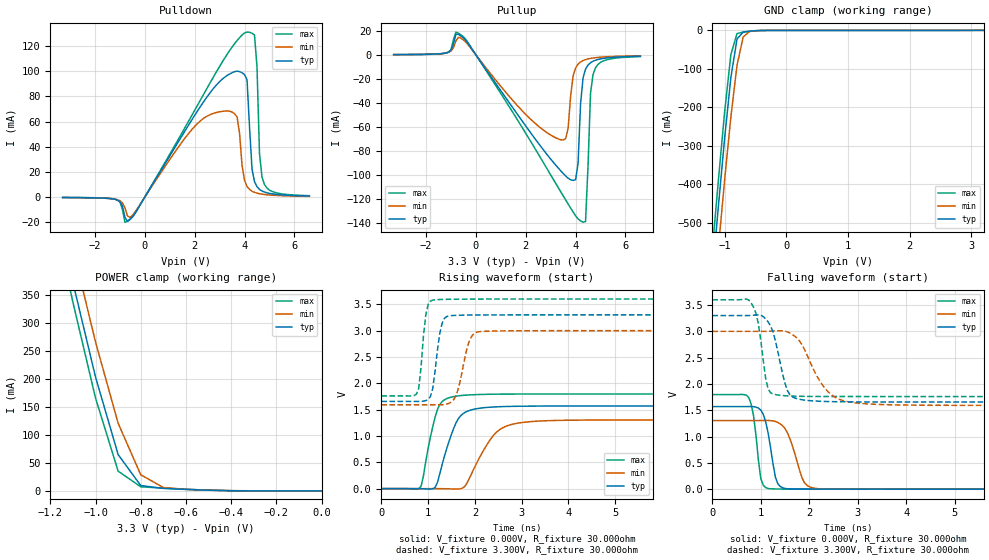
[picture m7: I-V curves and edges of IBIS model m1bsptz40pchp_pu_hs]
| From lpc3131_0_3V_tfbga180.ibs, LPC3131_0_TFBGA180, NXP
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| |   Rev 0.20 IBIS Model Design Automation Generation   |
| |   N O N - S I L I C O N   C O R R E L A T E D   |
| |   This IBIS [Model] is pre-Beta tactical support   |
| |  Note: this IBIS [Model] contains clamp curves generated   |
| |   through simulation which should not be relied upon   |
| Date/Time   : 2010 Jan 25 (Mon) 11:58:19
| Pccmos090 jliolib_p50 2.0
|   0.9 um 3.3V pad library
|   seven level metal
|   dual oxide
|   dual threshold voltage
|   nominal line mixed supply
|   parasitic extracted netlists
| Process block a10
| mem1bsptz40pchp
|   Bidirectional Pad 3.3
|   3state Output
|   Plain Input
|   CMOS
|   Programmable between
|   - (p1=0, p2=1) plain input
|   - (p1=0, p2=0) with Pull Up
|   - (p1=1, p2=1) with Pull Down
|   - (p1=1, p2=0) with Repeater
| Pull Up Mode high speed (esh=0, p1=0, p2=0)
[Model]   m1bsptz40pchp_pu_hs | of mem1bsptz40pchp
Model_type   I/O
Polarity   Non-Inverting
Enable   Active-Low
|  Reciever Thresholds
Vinl   = 0.99V
Vinh   = 2.31V
| AC Test Load Conditions
Vref   = 0
Cref   = 0
Rref   = 1000000000
Vmeas   = 1.65
| [Process Range]   typical   min   max
| C_comp edge width   400.000ps   400.000ps   400.000ps
| C_comp Tstrobe   40.000fs   40.000fs   40.000fs
C_comp   200.000pF   200.000pF   200.000pF
[Temperature Range]   25   125   -40
[Voltage Range]   3.30V   3.00V   3.60V
[GND Clamp Reference]   0.00V   0.00V   0.00V
[Pulldown Reference]   0.00V   0.00V   0.00V
[POWER Clamp Reference]   3.30V   3.00V   3.60V
[Pullup Reference]   3.30V   3.00V   3.60V
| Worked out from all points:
|   slope of the pulldown table from 0 to 0.495 V, typ, clamps not added: 30.7 ohm
|   slope of the pullup table from 0 to 0.495 V, typ, clamps not added: 33.4 ohm
|   GND clamp passes 1 mA (typ) near -0.51 V on its own axis
|   POWER clamp passes 1 mA (typ) near -0.47 V on its own axis
|   rising waveform, V_fixture 0.000V, R_fixture 30.000ohm: 20-80 % time 341ps typ, 514ps min, 255ps max; typ from 0.001 V to 1.57 V
|   falling waveform, V_fixture 0.000V, R_fixture 30.000ohm: 20-80 % time 178ps typ, 272ps min, 137ps max; typ from 1.57 V to 0.001 V
|   rising waveform, V_fixture 3.300V, R_fixture 30.000ohm: 20-80 % time 144ps typ, 213ps min, 115ps max; typ from 1.66 V to 3.3 V
|   falling waveform, V_fixture 3.300V, R_fixture 30.000ohm: 20-80 % time 251ps typ, 501ps min, 169ps max; typ from 3.3 V to 1.66 V
[GND Clamp]
| ref voltage   0.00V   0.00V   0.00V
|   Voltage   I(typ)   I(min)   I(max)
-3.3V     -4.732A    -4.814A    -4.684A
-1.2V     -636mA     -742.5mA   -569.7mA
-1.1V     -453.5mA   -561.8mA   -385.7mA
-1V       -279mA     -387.5mA   -210.8mA
-900mV    -122.8mA   -225.5mA   -63.15mA
-800mV    -22.47mA   -90.5mA    -8.27mA
-700mV    -4.437mA   -17.32mA   -4.624mA
-600mV    -2.227mA   -3.085mA   -2.65mA
-300mV    -253.1uA   -168.6uA   -385.4uA
3.2V      -17.82uA   34.39uA    -87.56uA
[Power Clamp]   | Vtable = Vcc - Vpad
| ref voltage   3.30V   3.00V   3.60V
|   Voltage   I(typ)   I(min)   I(max)
-3.3V     4.647A     4.675A     4.636A
-1.2V     553.3mA    610.4mA    520.8mA
-1.1V     373.2mA    433.6mA    337.9mA
-1V       204mA      266.6mA    166.4mA
-900mV    65.07mA    121.2mA    35.4mA
-800mV    9.632mA    28.93mA    7.456mA
-700mV    4.576mA    6.079mA    4.901mA
-600mV    2.711mA    2.826mA    2.897mA
-400mV    366.5uA    549.1uA    304.5uA
0V        388.1pA    9.875nA    264.4pA
[Pulldown]
| ref voltage   0.00V   0.00V   0.00V
|   Voltage   I(typ)   I(min)   I(max)
-3.3V     -237uA     -253uA     -192.2uA
-1.2V     -1.654mA   -1.559mA   -1.497mA
-600mV    -17.52mA   -16.02mA   -17.7mA
2.8V      87.36mA    66.79mA    96.99mA
3.7V      99.96mA    63.73mA    124.2mA
4.1V      93mA       8.514mA    130.9mA
4.3V      22.4mA     4.741mA    130.1mA
4.4V      12.38mA    3.859mA    128.6mA
4.5V      8.362mA    3.243mA    103.4mA
4.6V      6.217mA    2.791mA    34.69mA
4.8V      4.107mA    2.175mA    10.04mA
6.6V      975.1uA    710.1uA    1.215mA
[Pullup]   | Vtable = Vcc - Vpad
| ref voltage   3.30V   3.00V   3.60V
|   Voltage   I(typ)   I(min)   I(max)
-3.3V     206.8uA    209.1uA    174.1uA
-500mV    14.05mA    12.42mA    15mA
3.4V      -96.4mA    -70.68mA   -113.8mA
3.7V      -102.7mA   -61.31mA   -124.1mA
3.9V      -104.5mA   -17.66mA   -130.8mA
4.1V      -90.31mA   -7.691mA   -136.5mA
4.2V      -40.65mA   -5.885mA   -138.2mA
4.3V      -19.22mA   -4.74mA    -139.3mA
4.4V      -11.93mA   -3.955mA   -138.7mA
4.6V      -6.527mA   -2.958mA   -31.83mA
4.7V      -5.3mA     -2.623mA   -16.4mA
6.6V      -1.122mA   -812.7uA   -1.418mA
[Ramp]
R_load   = 30.000ohm
|   dV/dt(typ)   dV/dt(min)   dV/dt(max)
dV/dt_r   941.416mV/350.000ps   782.862mV/500.000ps   1.078V/250.000ps
dV/dt_f   985.623mV/250.000ps   844.107mV/500.000ps   1.103V/150.000ps
[Rising Waveform]  | cubic spline decimation from 501 points
V_fixture   = 0.000V
R_fixture   = 30.000ohm
|   Time   V(typ)   V(min)   V(max)
0s        906.1uV    713.4uV    1.177mV
850ps     -657.1uV   736.3uV    46.19mV
1.15ns    25.24mV    854.7uV    1.359V
1.3ns     457.5mV    -208.2uV   1.654V
1.55ns    1.154V     -5.889mV   1.749V
1.8ns     1.454V     61.17mV    1.776V
2.2ns     1.538V     751mV      1.79V
2.45ns    1.553V     1.063V     1.794V
3.3ns     1.568V     1.28V      1.797V
25ns      1.57V      1.305V     1.798V
[Falling Waveform]  | cubic spline decimation from 501 points
V_fixture   = 0.000V
R_fixture   = 30.000ohm
|   Time   V(typ)   V(min)   V(max)
0s        1.57V      1.305V     1.798V
750ps     1.571V     1.305V     1.742V
850ps     1.569V     1.305V     1.395V
1ns       1.504V     1.306V     198.2mV
1.2ns     794.7mV    1.304V     7.889mV
1.3ns     230.7mV    1.287V     5.057mV
1.4ns     53.05mV    1.243V     3.511mV
1.9ns     2.346mV    124.6mV    1.427mV
2.2ns     1.395mV    8.421mV    1.267mV
25ns      906.1uV    713.5uV    1.177mV
[Rising Waveform]  | cubic spline decimation from 501 points
V_fixture   = 3.300V
V_fixture_min = 3.000V
V_fixture_max = 3.600V
R_fixture   = 30.000ohm
|   Time   V(typ)   V(min)   V(max)
0s        1.657V     1.593V     1.761V
750ps     1.657V     1.593V     1.794V
800ps     1.656V     1.593V     1.908V
950ps     1.672V     1.593V     3.295V
1.15ns    2.24V      1.592V     3.586V
1.35ns    3.235V     1.598V     3.594V
1.6ns     3.291V     1.776V     3.597V
1.9ns     3.297V     2.846V     3.599V
2.15ns    3.298V     2.985V     3.599V
25ns      3.3V       3V         3.6V
[Falling Waveform]  | cubic spline decimation from 501 points
V_fixture   = 3.300V
V_fixture_min = 3.000V
V_fixture_max = 3.600V
R_fixture   = 30.000ohm
|   Time   V(typ)   V(min)   V(max)
0s        3.3V       3V         3.6V
800ps     3.303V     3V         3.54V
950ps     3.313V     3V         3.141V
1.15ns    3.181V     3.002V     1.906V
1.25ns    2.993V     3.006V     1.81V
1.45ns    2.188V     3.009V     1.78V
1.7ns     1.735V     2.908V     1.768V
2.4ns     1.666V     1.842V     1.762V
3.1ns     1.659V     1.628V     1.761V
25ns      1.657V     1.593V     1.761V
